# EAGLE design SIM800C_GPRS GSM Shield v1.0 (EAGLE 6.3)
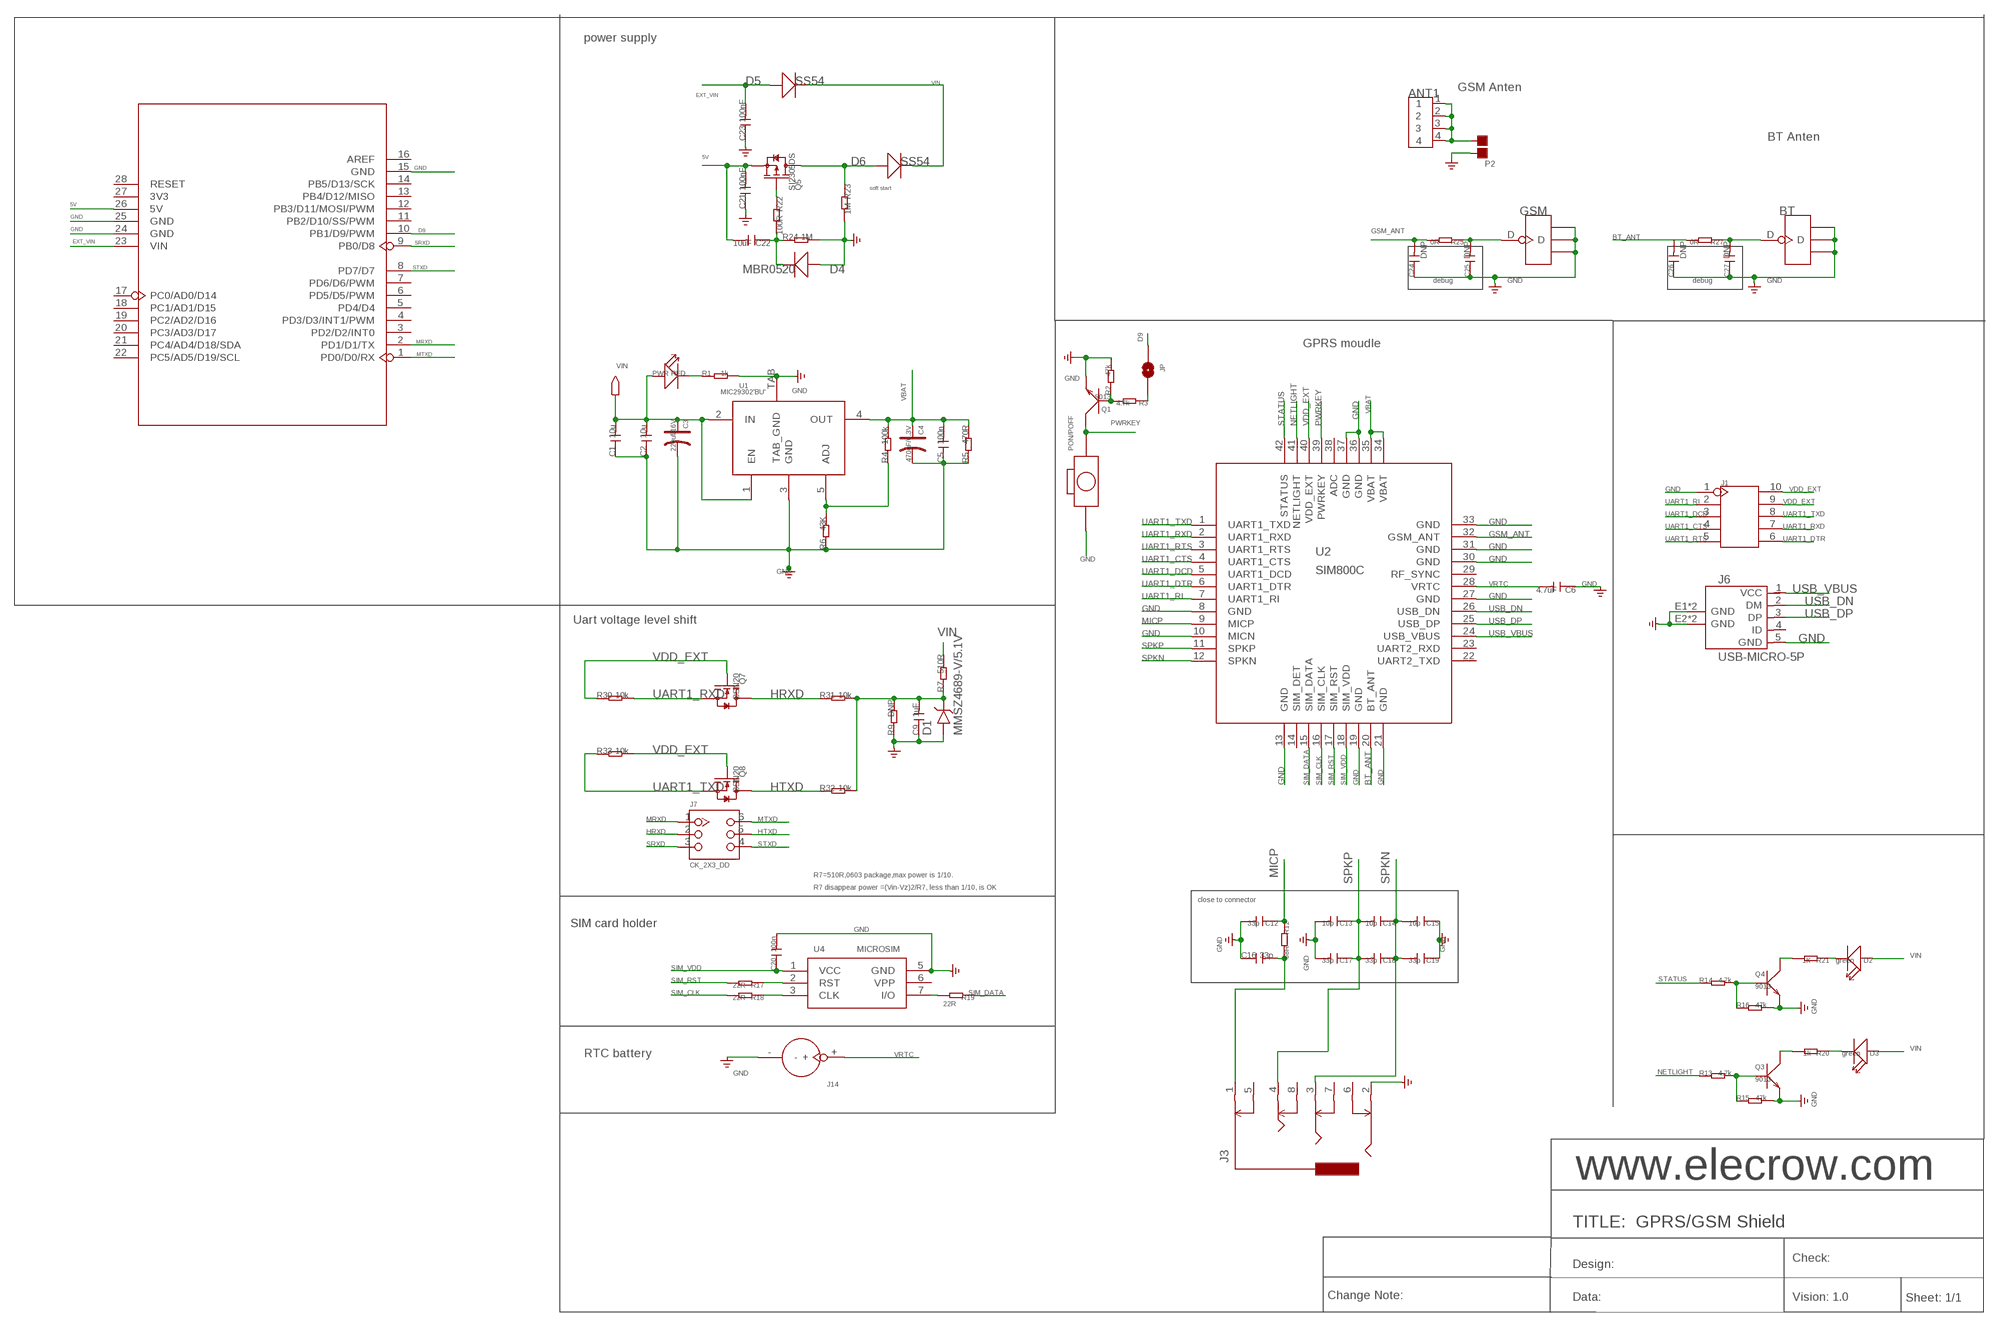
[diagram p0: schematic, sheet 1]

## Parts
ANT1  ANTENNA-SMA-IPX  [SMA-TO-IPX]
BT  ANTENNA-U-FL  [4P-U-FL]
C1  10u  C-0603  [C0603]
C2  10u  C-0603  [C0603]
C3  220uf/16V  006-CAP_AVX_D  [AVX_D]
C4  470uF/6.3V  006-CAP_AVX_D  [AVX_D]
C5  100n  C-0603  [C0603]
C6  4.7uF  C-0805  [C0805]
C9  1uF  C-0603  [C0603]
C12  33p  C-0603  [C0603]
C13  10p  C-0402  [C0402]
C14  10p  C-0402  [C0402]
C15  10p  C-0402  [C0402]
C16  33p  C-0603  [C0603]
C17  33p  C-0402  [C0402]
C18  33p  C-0402  [C0402]
C19  33p  C-0402  [C0402]
C20  100n  C-0603  [C0603]
C21  100nF  C-0603  [C0603]
C22  10uF  C-0805  [C0805]
C23  100nF  C-0603  [C0603]
C24  DNP  C-0402  [C0402]
C25  DNP  C-0402  [C0402]
C26  DNP  C-0402  [C0402]
C27  DNP  C-0402  [C0402]
D1  MMSZ4689-V/5.1V  D-VOL'MMSZ4681'  [SOD123-2.7X1.6]
D2  green  LED'0603'  [LED-0603]
D3  green  LED'0603'  [LED-0603]
D4  MBR0520  D'MBR0520LT1'  [SOD123-2.7X1.6]
D5  SS54  D'MBRS240LT3'  [SMB]
D6  SS54  D'MBRS240LT3'  [SMB]
GSM  ANTENNA-U-FL  [4P-U-FL]
J1  HEADER-2X5P-2.54  [2X5P-2.54]
J3  AUDIO-8P'PJ-3536-L6S'  [8P-3.5-SMD]
J6  USB-MICRO-5P  [MICRO-USB-5P]
J7  CK_2X3_DD  [CK_2X3]
J14  HOLDER-BATTERY-2P-CR1220  [CR1220]
JP  0R/0805  PAD-SOLDERJUMPERNC  [2P-SMD-3.3X2]
P2  PAD-JUMPER-2P  [2P-SMD-1.78X1.27]
PON/POFF  BOTTON_1_DP  [BTN_5.0_RST]
PWR  RED  007-LED0603  [D0603]
Q1  9013  TRANSISTOR-NPN-SOT23  [SOT23]
Q3  9013  TRANSISTOR-NPN-SOT23  [SOT23]
Q4  9013  TRANSISTOR-NPN-SOT23  [SOT23]
Q5  SI2305DS  MOSFET-P'SI2323CDS/SI2305DS<BR>'  [SOT23]
Q7  BSN20  MOSFET-N'SOT23'  [SOT23]
Q8  BSN20  MOSFET-N'SOT23'  [SOT23]
R1  1k  R-0603  [R0603]
R2  47k  R-0603  [R0603]
R3  4.7k  R-0603  [R0603]
R4  100k  R-0603  [R0603]
R5  470R  R-0603  [R0603]
R6  43K  R-0603  [R0603]
R7  510R  R-0603  [R0603]
R9  DNP  R-0603  [R0603]
R12  68R  R-0603  [R0603]
R13  4.7k  R-0603  [R0603]
R14  4.7k  R-0603  [R0603]
R15  47k  R-0603  [R0603]
R16  47k  R-0603  [R0603]
R17  22R  R-0603  [R0603]
R18  22R  R-0603  [R0603]
R19  22R  R-0603  [R0603]
R20  1k  R-0603  [R0603]
R21  1K  R-0603  [R0603]
R22  100R  R-0603  [R0603]
R23  1M  R-0603  [R0603]
R24  1M  R-0603  [R0603]
R25  0R  R-0402  [R0402]
R27  0R  R-0402  [R0402]
R30  10k  R-0603  [R0603]
R31  10k  R-0603  [R0603]
R32  10k  R-0603  [R0603]
R33  10k  R-0603  [R0603]
U1  MIC29302'BU'  [TO-263]
U2  SIM800C  [SIM800C]
U3  UNO-SHILED  [SHILED]
U4  MICROSIM  [MICROSIM]

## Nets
5V: C21.2 C22.2 Q5.2(S) U3.26(5V)
BT_ANT: C26.2 R27.2 U2.20(BT_ANT)
D9: JP.1 U3.10(PB1/D9/PWM)
EXT_VIN: C23.2 D5.+ U3.23(VIN)
GND: BT.GND1 BT.GND2 BT.GND3 C1.1 C2.1 C3.- C4.- C5.1 C6.1 C9.1 C12.2 C13.2 C15.1 C16.1 C17.2 C19.1 C20.2 C21.1 C23.1 C24.1 C25.1 C26.1 C27.1 D1.1 D4.1(+) GSM.GND1 GSM.GND2 GSM.GND3 J1.1 J3.2 J6.5(GND) J6.E1(GND) J6.E2(GND) J6.P1(GND) J6.P2(GND) J14.- P2.2 PON/POFF.P$1 Q1.2(E) Q3.2(E) Q4.2(E) R1.2 R2.2 R5.1 R6.1 R9.1 R15.2 R16.2 R23.2 R24.2 U1.3(GND) U1.TAB(TAB_GND) U2.8(GND) U2.10(MICN) U2.13(GND) U2.19(GND) U2.21(GND) U2.27(GND) U2.30(GND) U2.31(GND) U2.33(GND) U2.36(GND) U2.37(GND) U3.15(GND) U3.24(GND) U3.25(GND) U4.5(GND)
GSM_ANT: C24.2 R25.2 U2.32(GSM_ANT)
HRXD: J7.2 Q7.3(D) R31.1
HTXD: J7.5 Q8.3(D) R32.1
MICP: C12.1 R12.1 U2.9(MICP)
MRXD: J7.1 U3.2(PD1/D1/TX)
MTXD: J7.6 U3.1(PD0/D0/RX)
N$1: R19.2 U4.7(I/O)
N$2: R4.1 R6.2 U1.5(ADJ)
N$3: Q3.3(C) R20.2
N$5: R18.1 U4.3(CLK)
N$6: R17.1 U4.2(RST)
N$7: D3.- R20.1
N$8: Q3.1(B) R13.2 R15.1
N$9: C9.2 D1.2 R7.1 R9.2 R31.2 R32.2
N$11: Q5.1(G) R22.1
N$12: ANT1.1 ANT1.2 ANT1.3 ANT1.4 P2.1
N$14: JP.2 R3.1
N$16: Q4.3(C) R21.2
N$17: D2.- R21.1
N$18: Q4.1(B) R14.2 R16.1
N$20: D6.+ Q5.3(D) R23.1
N$25: C25.2 GSM.D R25.1
N$28: BT.D C27.2 R27.1
N$30: C16.2 J3.1 R12.2
N$36: Q1.1(B) R2.1 R3.2
N$39: C22.1 D4.2(-) R22.2 R24.1
N$53: PWR.- R1.1
NETLIGHT: R13.1 U2.41(NETLIGHT)
PWRKEY: PON/POFF.P$2 Q1.3(C) U2.39(PWRKEY)
SIM_CLK: R18.2 U2.16(SIM_CLK)
SIM_DATA: R19.1 U2.15(SIM_DATA)
SIM_RST: R17.2 U2.17(SIM_RST)
SIM_VDD: C20.1 U2.18(SIM_VDD) U4.1(VCC)
SPKN: C14.1 C15.2 C18.1 C19.2 J3.3 U2.12(SPKN)
SPKP: C13.1 C14.2 C17.1 C18.2 J3.4 U2.11(SPKP)
SRXD: J7.3 U3.9(PB0/D8)
STATUS: R14.1 U2.42(STATUS)
STXD: J7.4 U3.8(PD7/D7)
UART1_CTS: J1.4 U2.4(UART1_CTS)
UART1_DCD: J1.3 U2.5(UART1_DCD)
UART1_DTR: J1.6 U2.6(UART1_DTR)
UART1_RI: J1.2 U2.7(UART1_RI)
UART1_RTS: J1.5 U2.3(UART1_RTS)
UART1_RXD: J1.7 Q7.2(S) R30.2 U2.2(UART1_RXD)
UART1_TXD: J1.8 Q8.2(S) R33.1 U2.1(UART1_TXD)
USB_DN: J6.2(DM) U2.26(USB_DN)
USB_DP: J6.3(DP) U2.25(USB_DP)
USB_VBUS: J6.1(VCC) U2.24(USB_VBUS)
VBAT: C4.+ C5.2 R4.2 R5.2 U1.4(OUT) U2.34(VBAT) U2.35(VBAT)
VDD_EXT: J1.9 J1.10 Q7.1(G) Q8.1(G) R30.1 R33.2 U2.40(VDD_EXT)
VIN: C1.2 C2.2 C3.+ D2.+ D3.+ D5.- D6.- PWR.+ R7.2 U1.1(EN) U1.2(IN)
VRTC: C6.2 J14.+ U2.28(VRTC)
Unconnected: J3.5 J3.6 J3.7 J3.8 J6.4(ID) U2.14(SIM_DET) U2.22(UART2_TXD) U2.23(UART2_RXD) U2.29(RF_SYNC) U2.38(ADC) U3.3(PD2/D2/INT0) U3.4(PD3/D3/INT1/PWM) U3.5(PD4/D4) U3.6(PD5/D5/PWM) U3.7(PD6/D6/PWM) U3.11(PB2/D10/SS/PWM) U3.12(PB3/D11/MOSI/PWM) U3.13(PB4/D12/MISO) U3.14(PB5/D13/SCK) U3.16(AREF) U3.17(PC0/AD0/D14) U3.18(PC1/AD1/D15) U3.19(PC2/AD2/D16) U3.20(PC3/AD3/D17) U3.21(PC4/AD4/D18/SDA) U3.22(PC5/AD5/D19/SCL) U3.27(3V3) U3.28(RESET) U4.6(VPP)

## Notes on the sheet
- power supply
- GSM Anten
- BT Anten
- soft start
- debug | debug
- GPRS moudle
- Uart voltage level shift
- R7=510R,0603 package,max power is 1/10.
- R7 disappear power =(Vin-Vz)2/R7, less than 1/10, is OK
- close to connector
- SIM card holder
- RTC battery
- www.elecrow.com
- TITLE:  GPRS/GSM Shield
- Check:
- Design:
- Change Note: | Data: | Vision: 1.0 | Sheet: 1/1

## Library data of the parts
ANT1 = Connector:ANTENNA-SMA-IPX
BT GSM = Connector:ANTENNA-U-FL
C1 C2 C5 C6 C9 C12-C27 = Discrete:C*: Ceramic Capacitors
C3 C4 = Discrete:006-CAP*: Electrolytic Capacitors,Tantalum Capacitors and Super Capacitors
D1 = template:D-VOL
D2 D3 = Discrete:LED*
D4-D6 = Discrete:D*
J1 = Connector:HEADER-2X5P
J3 = template:AUDIO-8P
J6 = Connector:USB-MICRO-5P
J7 = CONNECTER:CK_2X3
J14 = Connector:HOLDER-BATTERY-2P
JP = Discrete:PAD-SOLDERJUMPER: Solder Jumper
P2 = Discrete:PAD-JUMPER-2P; PARTNO: DNP
PON/POFF = CPT_SMD:BOTTON_1
PWR = Discrete:007-LED*
Q1 Q3 Q4 = Discrete:TRANSISTOR-NPN*: NPN audion
Q5 = Discrete:MOSFET-P
Q7 Q8 = Discrete:MOSFET-N: IRLL014: http://www.vishay.com/docs/91319/sihll014.pdf
R1-R7 R9 R12-R25 R27 R30-R33 = Discrete:R*
U1 = ICs_v54:MIC29302
U2 = moudle:SIM800C
U3 = ljb:UNO-SHILED
U4 = Connector:MICROSIM

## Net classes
0 default: width 0.152 mm, drill 0.152 mm, clearance 0.152 mm

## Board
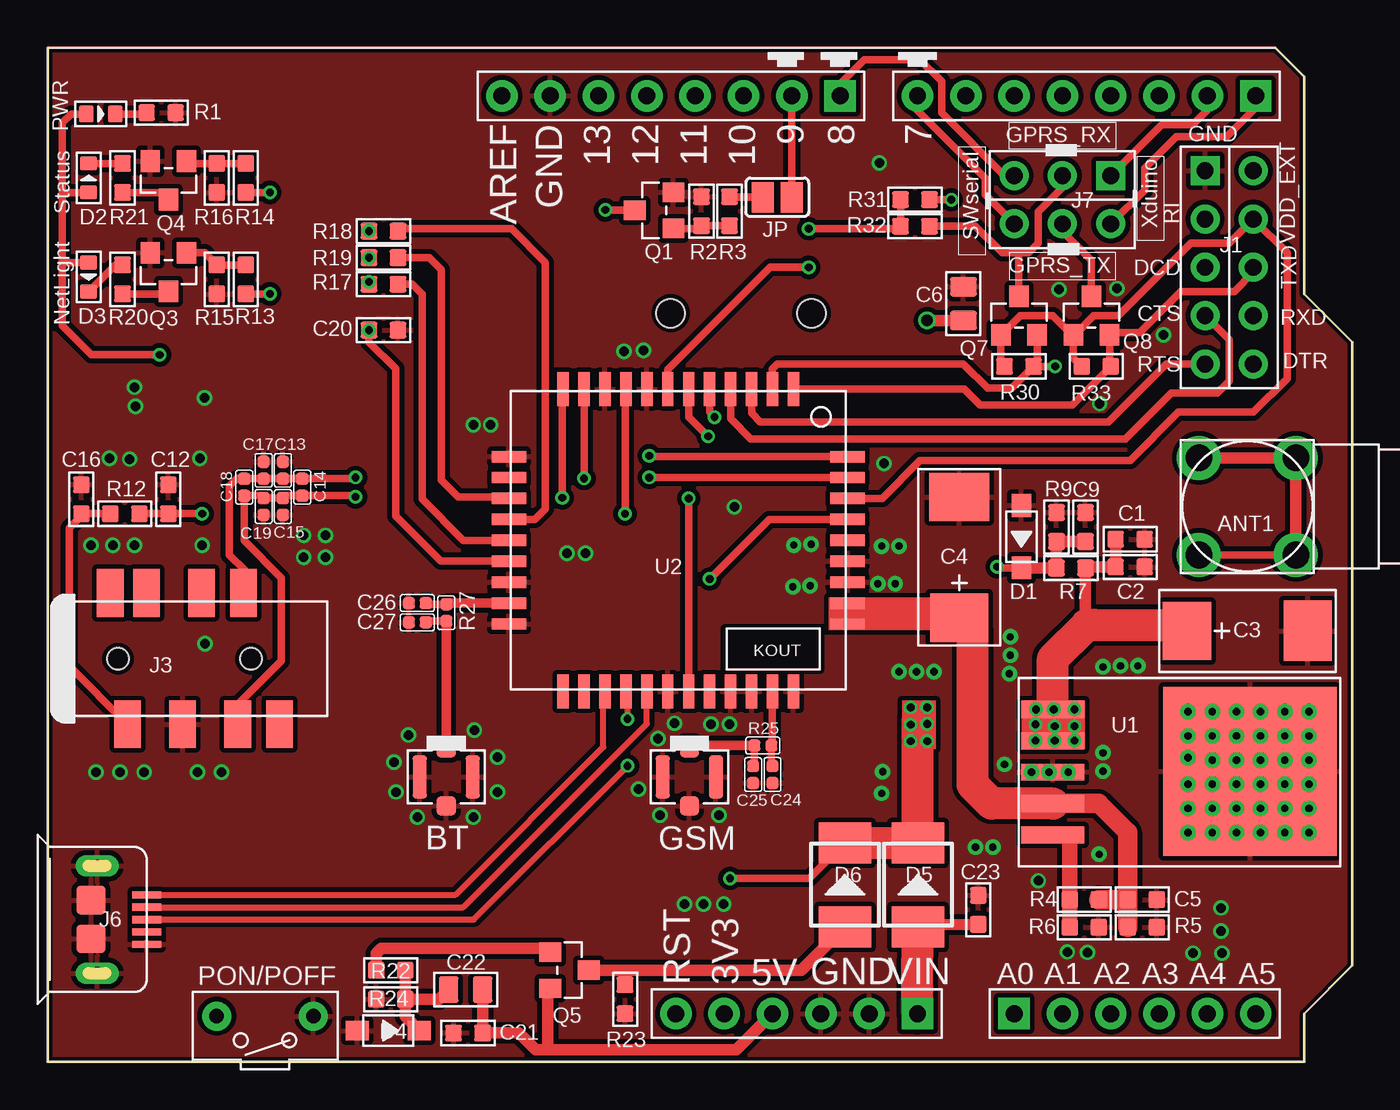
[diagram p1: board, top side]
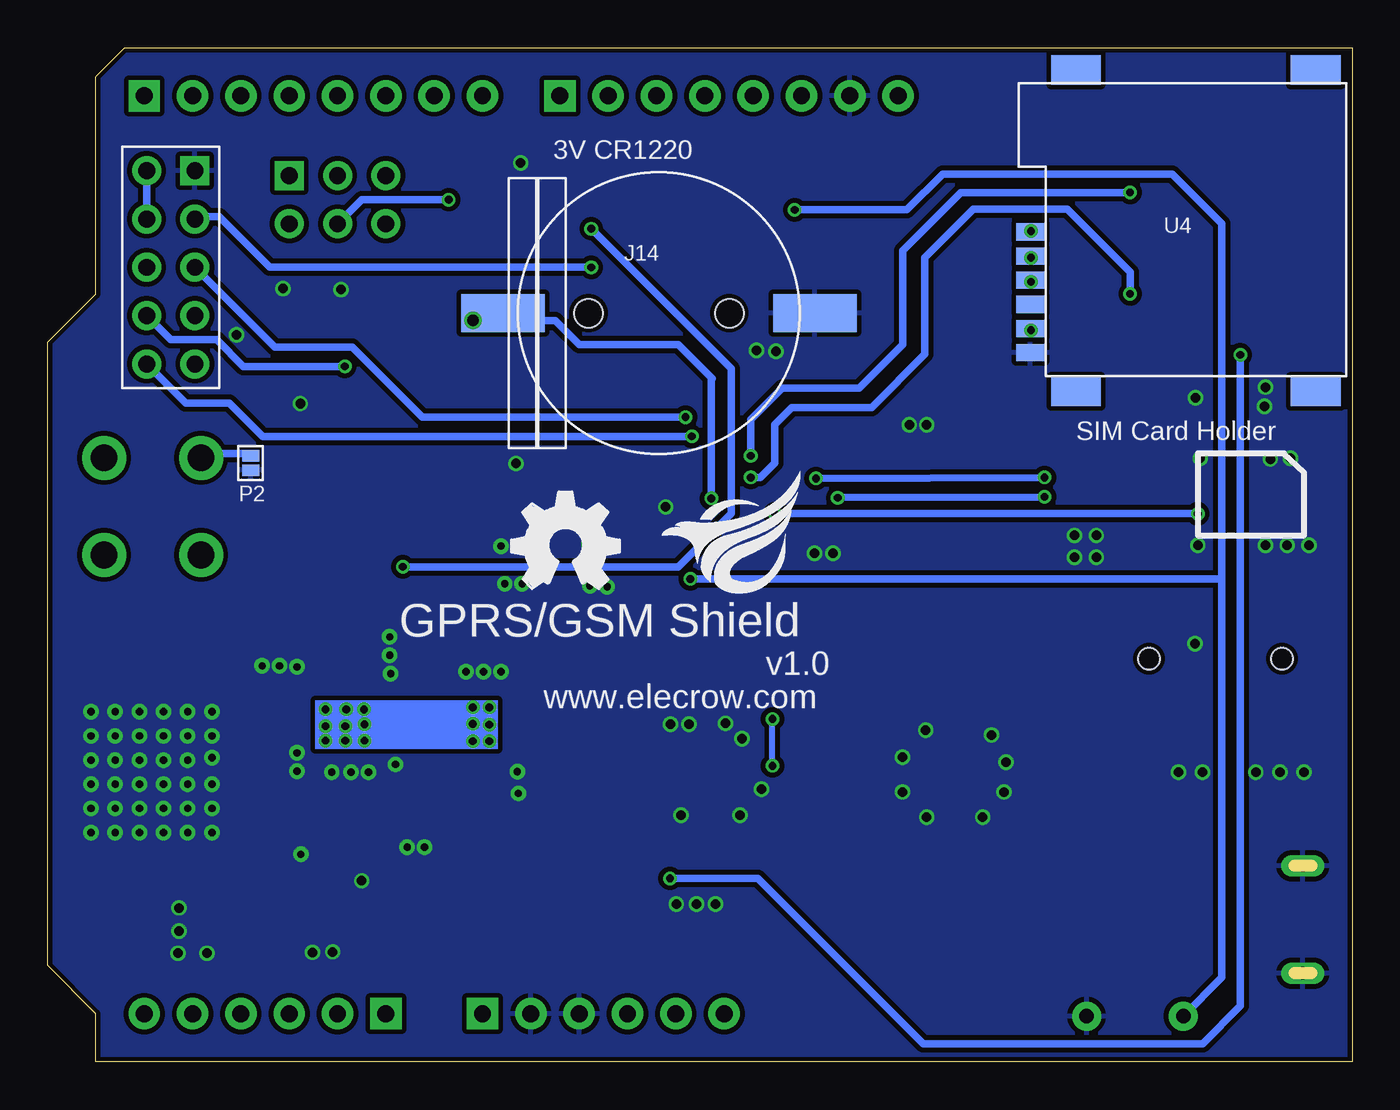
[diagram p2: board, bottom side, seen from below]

Size 68.58 x 53.34 mm. Coordinates in mm from the lower left corner, seen from the top.
Outline: 0,0 66.04,0 66.04,2.54 68.58,5.08 68.58,37.85 66.04,40.39 66.04,51.82 64.52,53.34 0,53.34 0,0
Copper layers (1*16): Top 0.035mm / dielectric 1.5mm / Bottom 0.035mm
Design rules "SeeedStudio_rule_no_angle_090911": minimum track width 6mil, minimum drill 12mil, track to track 6mil, track to pad 6mil, pad to pad 6mil, via to via 6mil, smd to smd 0mil, copper to edge 10mil, drill to drill 10mil, minimum pad ring 10mil, minimum via ring 6mil, stop-mask expansion 2mil, vias tented up to drill 100mil, thermal gap 10mil
tRestrict: 1 lines

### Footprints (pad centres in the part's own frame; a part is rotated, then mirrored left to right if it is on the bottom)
SMA-TO-IPX = drill 1.4 pad 2.3: 1 -2.55,2.55; 2 2.55,2.55; 3 2.55,-2.55; 4 -2.55,-2.55
4P-U-FL = smd 1.016 x 1.016: D -1.524,0; GND3 1.524,0 | smd 2.286 x 0.762: GND1 0,1.397; GND2 0,-1.397
C0603 = smd 0.889 x 0.889: 1 -0.762,0; 2 0.762,0
AVX_D = smd 2.54 x 3.048: + -3.175,0 | smd 2.54 x 3.175: - 3.175,0
C0805 = smd 1.016 x 1.397: 1 -0.889,0; 2 0.889,0
C0402 = smd 0.635 x 0.635: 1 -0.445,0; 2 0.445,0
SOD123-2.7X1.6 = smd 1.2 x 1.02: 1 -1.635,0; 2 1.635,0
D0603 = smd 0.762 x 0.889: + -0.762,0; - 0.762,0
SMB = smd 2.159 x 2.743: + -2.21,0; - 2.21,0
2X5P-2.54-LEADED = drill 0.889 pad 1.524 square: 1 -1.27,5.08 | drill 0.889 pad 1.524: 2 -1.27,2.54; 3 -1.27,0; 4 -1.27,-2.54; 5 -1.27,-5.08; 6 1.27,-5.08; 7 1.27,-2.54; 8 1.27,0; 9 1.27,2.54; 10 1.27,5.08
8P-3.5-SMD = smd 1.4 x 2.5: 1 2.8,-3.45; 2 5.7,-3.45; 3 8.6,-3.45; 4 8.9,3.45; 5 1.9,3.45; 6 3.8,3.45; 7 6.7,3.45; 8 10.8,-3.45 | hole 1.149: 2.3,0; 9.3,0
MICRO-USB-5P = smd 0.38 x 1.52: 1 -1.3,0; 2 -0.65,0; 3 0,0; 4 0.65,0; 5 1.3,0 | smd 1.524 x 1.524: E1 -1.016,-2.921; E2 1.016,-2.921 | drill 0.635 pad 1.143 long: P1 -2.819,-2.591; P2 2.819,-2.591
CK_2X3 = drill 0.889 pad 1.524 square: 1 -1.27,2.54 | drill 0.889 pad 1.524: 2 -1.27,0; 3 -1.27,-2.54; 4 1.27,-2.54; 5 1.27,0; 6 1.27,2.54
CR1220 = smd 2 x 4.4: + 0,-8.2; - 0,8.2 | hole 1.5: 0,3.7; 0,-3.7
2P-SMD-3.3X2 = smd 1.168 x 1.6: 1 -0.762,0; 2 0.762,0
2P-SMD-1.78X1.27 = smd 0.889 x 0.61: 1 0,0.381; 2 0,-0.381
BTN_5.0_RST = drill 0.762 pad 1.524: P$1 0,2.54; P$2 0,-2.54
SOT23 = smd 1.016 x 1.143: 1 -0.95,-1.016; 2 0.95,-1.016; 3 0,1.016
R0603 = smd 0.889 x 0.889: 1 -0.762,0; 2 0.762,0
R0402 = smd 0.635 x 0.635: 1 -0.445,0; 2 0.445,0
TO-263 = smd 3.302 x 0.889: 1 3.302,-3.302; 2 3.302,-1.651; 3 3.302,0; 4 3.302,1.651; 5 3.302,3.302 | smd 9.12 x 8.89: TAB -7.071,-0.03
SIM800C = smd 1.8 x 0.6: 1 -7.95,6.05; 2 -7.95,4.95; 3 -7.95,3.85; 4 -7.95,2.75; 5 -7.95,1.65; 6 -7.95,0.55; 7 -7.95,-0.55; 8 -7.95,-1.65; 9 -7.95,-2.75; 10 -7.95,-3.85; 11 -7.95,-4.95; 12 -7.95,-6.05; 22 7.95,-6.05; 23 7.95,-4.95; 24 7.95,-3.85; 25 7.95,-2.75; 26 7.95,-1.65; 27 7.95,-0.55; 28 7.95,0.55; 29 7.95,1.65; 30 7.95,2.75; 31 7.95,3.85; 32 7.95,4.95; 33 7.95,6.05 | smd 0.6 x 1.8: 13 -4.4,-8.9; 14 -3.3,-8.9; 15 -2.2,-8.9; 16 -1.1,-8.9; 17 0,-8.9; 18 1.1,-8.9; 19 2.2,-8.9; 20 3.3,-8.9; 21 4.4,-8.9; 34 4.4,8.9; 35 3.3,8.9; 36 2.2,8.9; 37 1.1,8.9; 38 0,8.9; 39 -1.1,8.9; 40 -2.2,8.9; 41 -3.3,8.9; 42 -4.4,8.9
SHILED = drill 0.889 pad 1.651 square: 1 63.5,50.8; 9 41.656,50.8; 17 50.8,2.54; 23 45.72,2.54 | drill 0.889 pad 1.651: 2 60.96,50.8; 3 58.42,50.8; 4 55.88,50.8; 5 53.34,50.8; 6 50.8,50.8; 7 48.26,50.8; 8 45.72,50.8; 10 39.116,50.8; 11 36.576,50.8; 12 34.036,50.8; 13 31.496,50.8; 14 28.956,50.8; 15 26.416,50.8; 16 23.876,50.8; 18 53.34,2.54; 19 55.88,2.54; 20 58.42,2.54; 21 60.96,2.54; 22 63.5,2.54; 24 43.18,2.54; 25 40.64,2.54; 26 38.1,2.54; 27 35.56,2.54; 28 33.02,2.54
MICROSIM = smd 1.5 x 0.9: 1 -0.8,2.5; 2 -0.8,5.04; 3 -0.8,7.58; 5 -0.8,1.23; 6 -0.8,3.77; 7 -0.8,6.31 | smd 2.61 x 1.56: P$1 1.6,-0.8; P$2 14.2,-0.8; P$3 14.2,16.1; P$4 1.6,16.1

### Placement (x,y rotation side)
ANT1  63.06,29.21 90 top
BT  20.95,14.99 270 top
C1  56.9,27.48 180 top
C2  56.9,26.04 180 top
C3  63.06,22.67 0 top
C4  47.92,26.53 90 top
C5  57.53,8.53 180 top
C6  48.13,39.88 270 top
C9  54.55,28.13 270 top
C12  6.35,29.59 90 top
C13  12.37,31.11 90 top
C14  13.39,30.23 90 top
C15  12.37,29.21 90 top
C16  1.78,29.59 270 top
C17  11.35,31.11 90 top
C18  10.34,30.23 90 top
C19  11.35,29.21 90 top
C20  17.65,38.48 0 top
C21  22.1,1.52 0 top
C22  21.97,3.81 0 top
C23  48.92,8 270 top
C24  38.1,15.11 90 top
C25  37.08,15.11 90 top
C26  19.43,24.13 0 top
C27  19.43,23.11 0 top
D1  51.18,27.62 270 top
D2  green  [D0603]  2.16,46.48 90 top
D3  green  [D0603]  2.16,41.27 270 top
D4  17.91,1.65 0 top
D5  45.75,9.32 90 top
D6  41.91,9.32 90 top
GSM  33.73,14.99 270 top
J1  [2X5P-2.54-LEADED]  62.1,41.78 0 top
J3  1.4,21.21 0 top
J6  5.21,7.49 270 top
J7  53.34,45.34 270 top
J14  36.45,39.37 270 bottom
JP  38.35,45.47 180 top
LOGO2  LOGO-OSHW-FILLX0200-NT  [OSHW_FILLX200_NOTEXT]  44.2,24.89 0 bottom
P2  57.91,31.5 0 bottom
PON/POFF  11.43,2.41 270 top
PWR  2.79,49.85 0 top
Q1  31.88,44.78 90 top
Q3  6.35,41.53 180 top
Q4  6.35,46.35 180 top
Q5  27.43,4.83 270 top
Q7  51.05,39.24 0 top
Q8  54.86,39.24 0 top
R1  5.97,49.91 0 top
R2  34.37,44.73 90 top
R3  35.84,44.73 270 top
R4  54.48,8.53 0 top
R5  57.53,7.09 180 top
R6  54.48,7.09 180 top
R7  53.78,25.97 0 top
R9  53.02,28.13 270 top
R12  4.06,28.83 180 top
R13  10.41,41.15 90 top
R14  10.41,46.48 90 top
R15  8.89,41.15 270 top
R16  8.89,46.48 270 top
R17  17.65,40.89 0 top
R18  17.65,43.69 0 top
R19  17.65,42.29 180 top
R20  3.94,41.15 270 top
R21  3.94,46.48 270 top
R22  18.03,4.83 0 top
R23  30.35,3.3 270 top
R24  18.03,3.3 180 top
R25  37.59,16.64 0 top
R27  20.95,23.62 90 top
R30  51.05,36.58 0 top
R31  45.59,43.94 180 top
R32  45.59,45.34 180 top
R33  55.12,36.58 180 top
U1  56.13,15.24 180 top
U2  33.15,27.43 270 top
U3  0,0 0 top
U4  16.13,36.07 0 bottom
U$4  [ELECROW_NRW_6]  36.32,24.64 0 bottom

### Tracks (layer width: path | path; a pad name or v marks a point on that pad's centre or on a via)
5V
  Top 0.61: C22.2 C21.2 24.77,1.52 25.65,0.64 26.29,0.64 | U3.26 36.2,0.64 26.29,0.64 | Q5.2 26.29,3.75 26.29,0.64
BT_ANT
  Top 0.406: 21.02,24.13 R27.2 19.94,24.07 C26.2
  Top 0.508: U2.20 21.02,24.13
D9
  Top 0.406: JP.1 U3.10
EXT_VIN
  Top 0.61: D5.+ 45.14,7.21 C23.2
  Top 1.676: U3.23 45.72,3.83 D5.+
GND  (via drill 0.38 pad 0.81, 0.5)
  other vias: 59.94,18.41 59.94,17.14 59.94,13.34 59.94,12.06 61.21,12.06 62.48,12.06 63.75,12.06 65.02,12.06 66.29,12.06 66.29,13.34 66.29,14.61 66.29,15.88 66.29,17.14 66.29,18.41 63.75,13.34 63.75,14.61 63.75,15.88 63.75,17.14 63.75,18.41 65.02,13.34 65.02,14.61 65.02,15.88 65.02,17.14 65.02,18.41 62.48,13.34 62.48,14.61 62.48,15.88 62.48,17.14 62.48,18.41 61.21,13.34 61.21,14.61 61.21,15.88 61.21,17.14 61.21,18.41 59.94,16 59.94,14.61 60.2,5.71 61.72,5.71 61.67,6.88 61.67,8.1 52.07,9.53 53.59,5.79 54.66,5.77 3.25,31.75 14.61,26.54 13.46,26.54 2.54,15.24 35.53,8.31 34.47,8.31 33.48,8.31 43.84,14.12 43.89,15.27 49.68,11.3 48.77,11.3 3.81,15.24 5.08,15.24 9.14,15.24 7.87,15.24 13.46,27.69 14.61,27.69 4.32,31.7 8,31.75 4.62,34.47 8.26,34.92 4.57,35.48 8.13,27.18 8.28,22 4.57,27.18 3.43,27.18 2.29,27.18 23.29,33.5 22.38,33.5 31.32,37.41 30.3,37.36 36.09,29.18 28.27,26.75 27.3,26.75 43.97,31.47 53.16,40.61 56.21,40.67 55.27,10.92 51.71,15.24 52.63,15.24 53.64,15.24 55.47,15.29 55.47,16.26 50.29,15.65 50.6,21.39 50.55,20.42 55.47,20.78 56.39,20.83 57.3,20.83 50.6,22.35 46.58,20.52 45.67,20.52 44.75,20.52 32.08,16.99 35.84,17.75 34.87,17.75 32.94,17.81 31.06,14.35 32.18,12.98 35.28,12.98 18.97,17.2 18.21,15.77 18.31,14.2 22.43,17.45 23.65,16.03 23.65,14.2 22.38,12.88 19.43,12.88 58.65,38.23 43.71,47.27 55.3,34.62 40.08,25.04 39.17,24.99 40.13,27.23 39.22,27.18 43.84,27.13 43.64,25.15 44.55,25.15 44.75,27.13
  pour Bottom (isolate 0.254): -1.27,-1.27 71.12,-1.27 71.12,54.61 -1.27,54.61
  pour Top (isolate 0.254): -1.27,-1.27 71.12,-1.27 71.12,54.61 -1.27,54.61
GSM_ANT
  Top 0.406: C24.2 38.04,15.62 R25.2 38.1,16.7 U2.32
HRXD
  Top 0.406: J7.2 53.34,45.97 52.07,44.7 52.07,43.05 51.56,42.55 51.05,42.55 | Q7.3 51.05,42.55 | 51.05,42.55 50.16,42.55 48.77,43.94 R31.1
HTXD  (via drill 0.41)
  Top 0.406: J7.5 53.34,43.69 54.86,42.16 Q8.3 | v47.5,45.34 R32.1
  Bottom 0.406: v47.5,45.34 52.07,45.34 J7.5
MICP  (via drill 0.41)
  Top 0.406: R12.1 C12.1 v8.13,28.83 | v30.35,28.83 30.35,35.24 U2.9
  Bottom 0.406: v8.13,28.83 v30.35,28.83
MRXD
  Top 0.406: J7.1 58.55,49.28 60.2,49.28 60.96,50.04 U3.2
MTXD
  Top 0.406: J7.6 57.66,45.85 57.66,46.99 59.31,48.64 61.98,48.64 63.5,50.16 U3.1
N$1  (via drill 0.41)
  Bottom 0.406: R19.2 16.84,42.29 U4.7
  other vias: 16.89,42.29
N$2
  Top 0.813: R6.2 R4.1 53.72,11.94 U1.5
N$3
  Top 0.406: Q3.3 6.22,40.39 R20.2
N$5  (via drill 0.41)
  Bottom 0.406: R18.1 U4.3
  other vias: 16.89,43.69
N$6  (via drill 0.41)
  Top 0.406: R17.1 v16.89,41.02
  Bottom 0.406: v16.89,41.02 16.89,41.15 U4.2
N$7
  Top 0.406: D3.- 3.56,41.91 R20.1
N$8
  Top 0.406: R13.2 R15.1 8.26,42.55 Q3.1
N$9  (via drill 0.41)
  Top 0.406: R32.2 R31.2 44.7,43.81 v40.01,43.81 | D1.2 49.96,25.99 v49.91,26.04
  Top 0.61: D1.2 53.01,25.99 R7.1 R9.2 C9.2
  Bottom 0.406: v49.91,26.04 35.43,26.04 32.64,28.83 32.64,36.45 v40.01,43.81
N$11
  Top 0.406: 26.22,5.97 Q5.1
  Top 0.61: R22.1 17.27,5.71 17.53,5.97 26.22,5.97
N$12
  Top 0.406: ANT1.1 ANT1.4
  Top 0.61: ANT1.4 ANT1.3 ANT1.2
  Bottom 0.406: P2.1 58.04,32 59.94,32 60.19,31.76 ANT1.2
N$14
  Top 0.406: JP.2 35.87,45.47 R3.1
N$16
  Top 0.406: Q4.3 5.97,45.72 R21.2
N$17
  Top 0.406: D2.- R21.1
N$18
  Top 0.406: Q4.1 7.43,47.24 R16.1 R14.2
N$20
  Top 0.61: Q5.3 30.35,4.83 | R23.1 30.35,4.83 | 30.35,4.83 39.62,4.83 D6.+
N$25
  Top 0.406: R25.1 37.15,15.62 C25.2
  Top 0.508: R25.1 33.86,16.64 GSM.D
N$28
  Top 0.406: R27.1 19.94,23.18 C27.2
  Top 0.508: R27.1 BT.D
N$30
  Top 0.406: C16.2 R12.2 3.04,28.57 | J3.1 1.14,20.81 1.14,28.07 1.78,28.7 C16.2 | 1.78,28.57 C16.2
N$36
  Top 0.406: Q1.1 34.23,43.83 R2.1 R3.2
N$39
  Top 0.61: R24.1 R22.2 | R24.1 20.57,3.3 C22.1 | D4.2 18.8,2.4 R24.1
N$53
  Top 0.406: PWR.- 5.21,49.85 R1.1
NETLIGHT  (via drill 0.41)
  Top 0.406: v11.68,40.39 R13.1 | U2.41 v31.62,30.73
  Bottom 0.406: v11.68,40.39 11.68,41.53 14.99,44.83 19.94,44.83 22.48,42.29 22.48,37.21 25.27,34.42 29.46,34.42 30.35,33.53 30.35,31.5 31.11,30.73 v31.62,30.73
PWRKEY  (via drill 0.41)
  Top 0.406: U2.39 37.93,28.53 v34.8,25.4 | Q1.3 29.34,44.78 v29.31,44.81
  Bottom 0.406: PON/POFF.P$2 6.86,4.45 6.86,25.53 | 6.86,25.53 6.86,44.07 9.47,46.69 21.54,46.69 23.42,44.81 v29.31,44.81 | v34.8,25.4 6.99,25.4 6.86,25.53
SIM_CLK
  Top 0.406: U2.16 25.61,28.53 26.16,29.08 26.16,42.04 24.38,43.81 18.54,43.81 R18.2
SIM_DATA
  Top 0.406: R19.1 20.07,42.29 20.7,41.66 20.7,30.61 21.59,29.72 24.26,29.72 U2.15
SIM_RST
  Top 0.406: R17.2 19.18,40.89 19.68,40.39 19.68,29.59 21.84,27.43 U2.17
SIM_VDD  (via drill 0.41)
  Top 0.406: U2.18 20.66,26.33 18.29,28.7 18.29,36.45 16.89,37.85 C20.1 16.76,38.61
  Bottom 0.406: U4.1 16.93,38.52 C20.1
  other vias: 16.89,38.48
SPKN  (via drill 0.41)
  Top 0.305: C15.2 12.5,29.78
  Top 0.406: C15.2 C19.2 11.23,29.78 C18.1 10.34,27.41 12.29,25.45 12.29,21.08 10.06,18.85 10.06,17.82 J3.3 | 12.5,29.78 C14.1 16.12,29.78 v16.18,29.72 | v27.05,29.67 27.05,35.24 U2.12
  Bottom 0.406: v16.18,29.72 v27.05,29.67
SPKP  (via drill 0.41)
  Top 0.406: v16.18,30.73 16.12,30.67 C14.2 C13.1 C17.1 C18.2 9.94,30.67 9.55,30.28 9.55,26.67 10.36,25.86 10.36,24.73 J3.4 | v28.19,30.68 28.19,35.28 U2.11
  Bottom 0.406: v16.18,30.73 v28.19,30.68
SRXD
  Top 0.406: J7.3 50.29,46.61 46.99,49.91 46.99,51.56 45.85,52.7 42.93,52.7 41.66,51.44 U3.9
STATUS  (via drill 0.41)
  Top 0.406: R14.1 v11.68,45.72 | U2.42 31.67,31.83 v31.62,31.88
  Bottom 0.406: v11.68,45.72 20.57,45.72 23.62,42.67 23.62,37.72 25.91,35.43 29.97,35.43 31.62,33.78 v31.62,31.88
STXD
  Top 0.406: J7.4 49.28,45.59 49.28,46.48 45.72,50.04 U3.8
UART1_CTS
  Top 0.406: U2.4 35.9,33.83 36.96,32.77 56.64,32.77 59.05,35.18 61.47,35.18 62.1,35.81 62.1,37.97 J1.4
UART1_DCD  (via drill 0.41)
  Top 0.406: U2.5 34.8,34.16 v35.05,33.91
  Bottom 0.406: v35.05,33.91 48.9,33.91 52.58,37.59 56.64,37.59 J1.3
UART1_DTR  (via drill 0.41)
  Top 0.406: U2.6 33.7,33.92 v34.72,32.89
  Bottom 0.406: v34.72,32.89 57.28,32.89 59.03,34.65 61.32,34.65 J1.6
UART1_RI  (via drill 0.41)
  Top 0.406: U2.7 32.6,36.41 37.97,41.78 v40.01,41.78
  Bottom 0.406: J1.2 60.71,44.45 59.56,44.45 56.9,41.78 v40.01,41.78
UART1_RTS
  Top 0.406: U2.3 37,34.12 37.47,33.66 55.75,33.66 58.8,36.7 J1.5
UART1_RXD  (via drill 0.41)
  Top 0.406: R30.2 52,36.76 Q7.2 | v52.96,36.58 R30.2 | U2.2 38.1,36.45 38.35,36.7 48.13,36.7 49.4,35.43 50.67,35.43 R30.2
  Bottom 0.406: v52.96,36.58 58.29,36.58 59.69,37.97 62.1,37.97 J1.7
UART1_TXD
  Top 0.406: J1.8 63.37,41.53 62.36,40.51 59.56,40.51 57.4,38.35 55.94,38.35 Q8.2 55.81,36.64 R33.1 53.85,34.54 49.02,34.54 48.18,35.38 U2.1
USB_DN
  Top 0.305: J6.2 21.86,8.14 31.5,17.78 31.5,19.58 U2.26
USB_DP  (via drill 0.41)
  Top 0.305: v30.48,18.03 30.48,19.5 U2.25 | J6.3 22.4,7.49 v30.48,15.57
  Bottom 0.305: v30.48,15.57 v30.48,18.03
USB_VBUS
  Top 0.305: J6.1 21.44,8.79 29.21,16.56 29.21,19.5 U2.24
VBAT
  Top 0.305: C4.+ 42.27,23.36 U2.34 U2.35
  Top 0.813: 56.77,9.14 56.77,9.02
  Top 1.016: R4.2 C5.2 | R5.2 C5.2 | U1.4 55.24,13.59 56.77,12.06 56.77,9.14 | 56.77,9.02 C5.2
  Top 1.676: U1.4 49.61,13.59 48.62,14.58 48.62,22.66 C4.+
VDD_EXT
  Top 0.406: R33.2 53.91,37.02 Q8.1 | Q8.1 53.85,38.23 52.83,39.24 51.12,39.24 Q7.1 50.1,36.76 R30.1 | Q8.1 53.98,38.23 54.99,39.24 56.26,39.24 60.07,43.05 62.1,43.05 J1.9 65.15,42.55 65.15,35.94 63.37,34.16 59.44,34.16 56.9,31.62 45.85,31.62 43.86,29.63 U2.40
  Bottom 0.406: J1.9 J1.10
VIN  (via drill 0.41)
  Top 0.305: 45.74,18.06 45.74,18.26 | 45.74,18.26 v45.36,18.64 | 45.74,18.26 45.95,18.26 | 45.95,18.26 v46.23,18.64 | 45.74,18.06 45.74,17.2 v45.36,16.87 v46.23,16.87 | 45.74,18.06 45.7,18.06 v45.36,17.73 | 45.95,18.26 45.95,18.06 v46.23,17.78 | v51.94,18.54 51.94,17.78 v51.92,17.75 v51.92,16.89
  Top 0.406: D2.+ 0.89,45.72 0.76,45.85 | PWR.+ 1.23,49.85 0.76,49.38 0.76,45.85 | 0.76,45.85 0.76,41.96 | 0.76,41.96 0.76,38.71 2.29,37.19 v5.89,37.19 | v51.94,18.54 U1.1 v52.88,18.54 v53.98,18.54 v53.98,17.65 | v53.98,17.65 v52.93,17.65 v52.93,16.89 U1.2 | v53.98,17.65 v53.98,16.89 | D3.+ 0.84,42.04 0.76,41.96 | v35.87,9.65 40.03,9.65 D6.-
  Top 0.61: C1.2 C2.2 54.61,26.04 R7.2 54.55,23.43 54.99,22.99
  Top 1.676: U1.1 52.83,21.21 54.61,22.99 54.99,22.99 59.56,22.99 C3.+ | D6.- D5.- 45.74,18.06
  Bottom 0.305: v45.36,18.64 51.84,18.64 v51.94,18.54
  Bottom 0.406: v5.89,37.19 5.89,2.95 7.87,0.96 22.55,0.96 31.24,9.65 v35.87,9.65
VRTC  (via drill 0.41, 0.61)
  Top 0.406: U2.28 v33.7,29.63
  Top 0.61: v46.23,38.99 C6.2
  Bottom 0.406: v46.23,38.99 41.91,38.99 40.64,37.72 35.43,37.72 33.7,35.98 | 33.7,35.98 33.66,35.94 | v33.7,29.63 33.7,35.98
  Bottom 0.61: J14.+ 45.03,38.99 v46.23,38.99
(copper drawn outside any net)
  shapes: Bottom area x1, Top area x3

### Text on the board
tPlace: 13 | 12 | 11 | 10 | 9 | 8 | 7 | GPRS_RX | SWserial | GND | VDD_EXT | Xduino | Status | RI | GPRS_TX | DCD | TXD | CTS | NetLight | RXD | RTS | DTR | RST | 3V3 | 5V | GND | VIN | A0 | A1 | A2 | A3 | A4 | A5
bPlace: 3V CR1220 | SIM Card Holder | GPRS/GSM Shield | v1.0 | www.elecrow.com
tNames: AREF | GND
